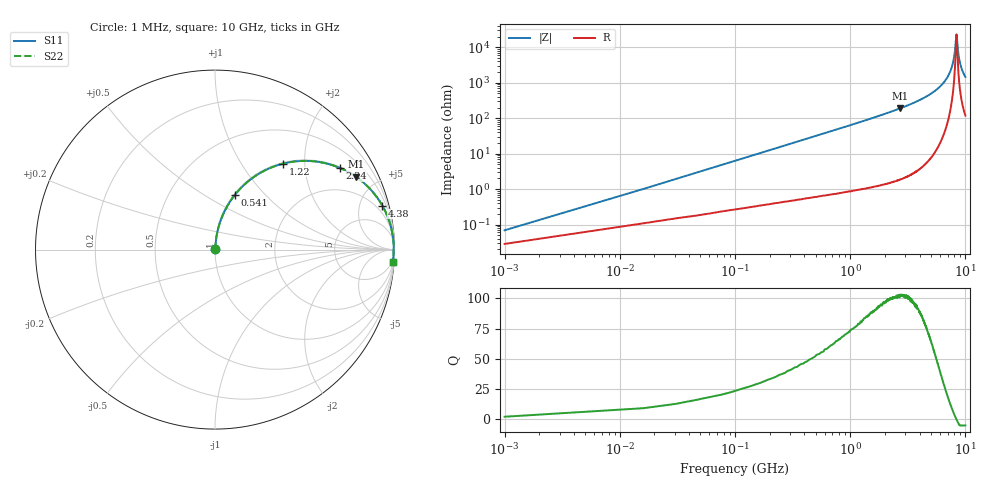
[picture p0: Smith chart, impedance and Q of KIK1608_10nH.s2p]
!version-2
!date-01.2022
!Series
# MHz S RI R 50
!Freq ReS11 ImS11 ReS21 ImS21 ReS12 ImS12 ReS22 ImS22
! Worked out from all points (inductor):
!   668 points, 1 MHz to 10 GHz, reference 50 ohm
!   read as one part in series: L = 10 nH near 46 MHz
!   highest Q = 102 at 2.73 GHz (marker M1), where L = 11.2 nH
!   self-resonance near 8.36 GHz
!   S11 on the Smith chart (normalised r, x): 1 MHz: 1.00, +0.00; 541 MHz: 1.01, +0.68; 1.22 GHz: 1.02, +1.56; 2.24 GHz: 1.03, +3.03; 4.38 GHz: 1.09, +7.59; 10 GHz: 3, -29
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1  0.000269 0.000628  0.9997 -0.000628  0.9997 -0.000628  0.000269 0.000628
61  0.00354 0.0381  0.9965 -0.0381  0.9965 -0.0381  0.00354 0.0381
121  0.00863 0.0752  0.9914 -0.0752  0.9914 -0.0752  0.00863 0.0752
286  0.0354 0.1728  0.9646 -0.1728  0.9646 -0.1728  0.0354 0.1728
541  0.1088 0.3023  0.8912 -0.3023  0.8912 -0.3023  0.1088 0.3023
1220  0.3801 0.4792  0.6199 -0.4792  0.6199 -0.4792  0.3801 0.4792
1670  0.5425 0.4927  0.4575 -0.4927  0.4575 -0.4927  0.5425 0.4927
2240  0.6942 0.4558  0.3058 -0.4558  0.3058 -0.4558  0.6942 0.4558
2730  0.7845 0.4063  0.2155 -0.4063  0.2155 -0.4063  0.7845 0.4063
3350  0.8598 0.3421  0.1402 -0.3421  0.1402 -0.3421  0.8598 0.3421
4380  0.9324 0.245  0.0676 -0.245  0.0676 -0.245  0.9324 0.245
5010  0.9574 0.1944  0.0426 -0.1944  0.0426 -0.1944  0.9574 0.1944
6680  0.9892 0.0853  0.0108 -0.0853  0.0108 -0.0853  0.9892 0.0853
7340  0.9938 0.0496  0.00618 -0.0496  0.00618 -0.0496  0.9938 0.0496
7790  0.9953 0.0271  0.00468 -0.0271  0.00468 -0.0271  0.9953 0.0271
8090  0.9957 0.0129  0.00429 -0.0129  0.00429 -0.0129  0.9957 0.0129
8340  0.9957 0.00114  0.00428 -0.00114  0.00428 -0.00114  0.9957 0.00114
8420  0.9957 -0.00223  0.00434 0.00223  0.00434 0.00223  0.9957 -0.00223
8670  0.9953 -0.0135  0.00469 0.0135  0.00469 0.0135  0.9953 -0.0135
8940  0.9947 -0.025  0.00533 0.025  0.00533 0.025  0.9947 -0.025
9390  0.993 -0.0435  0.00695 0.0435  0.00695 0.0435  0.993 -0.0435
10000  0.9899 -0.0671  0.0101 0.0671  0.0101 0.0671  0.9899 -0.0671
